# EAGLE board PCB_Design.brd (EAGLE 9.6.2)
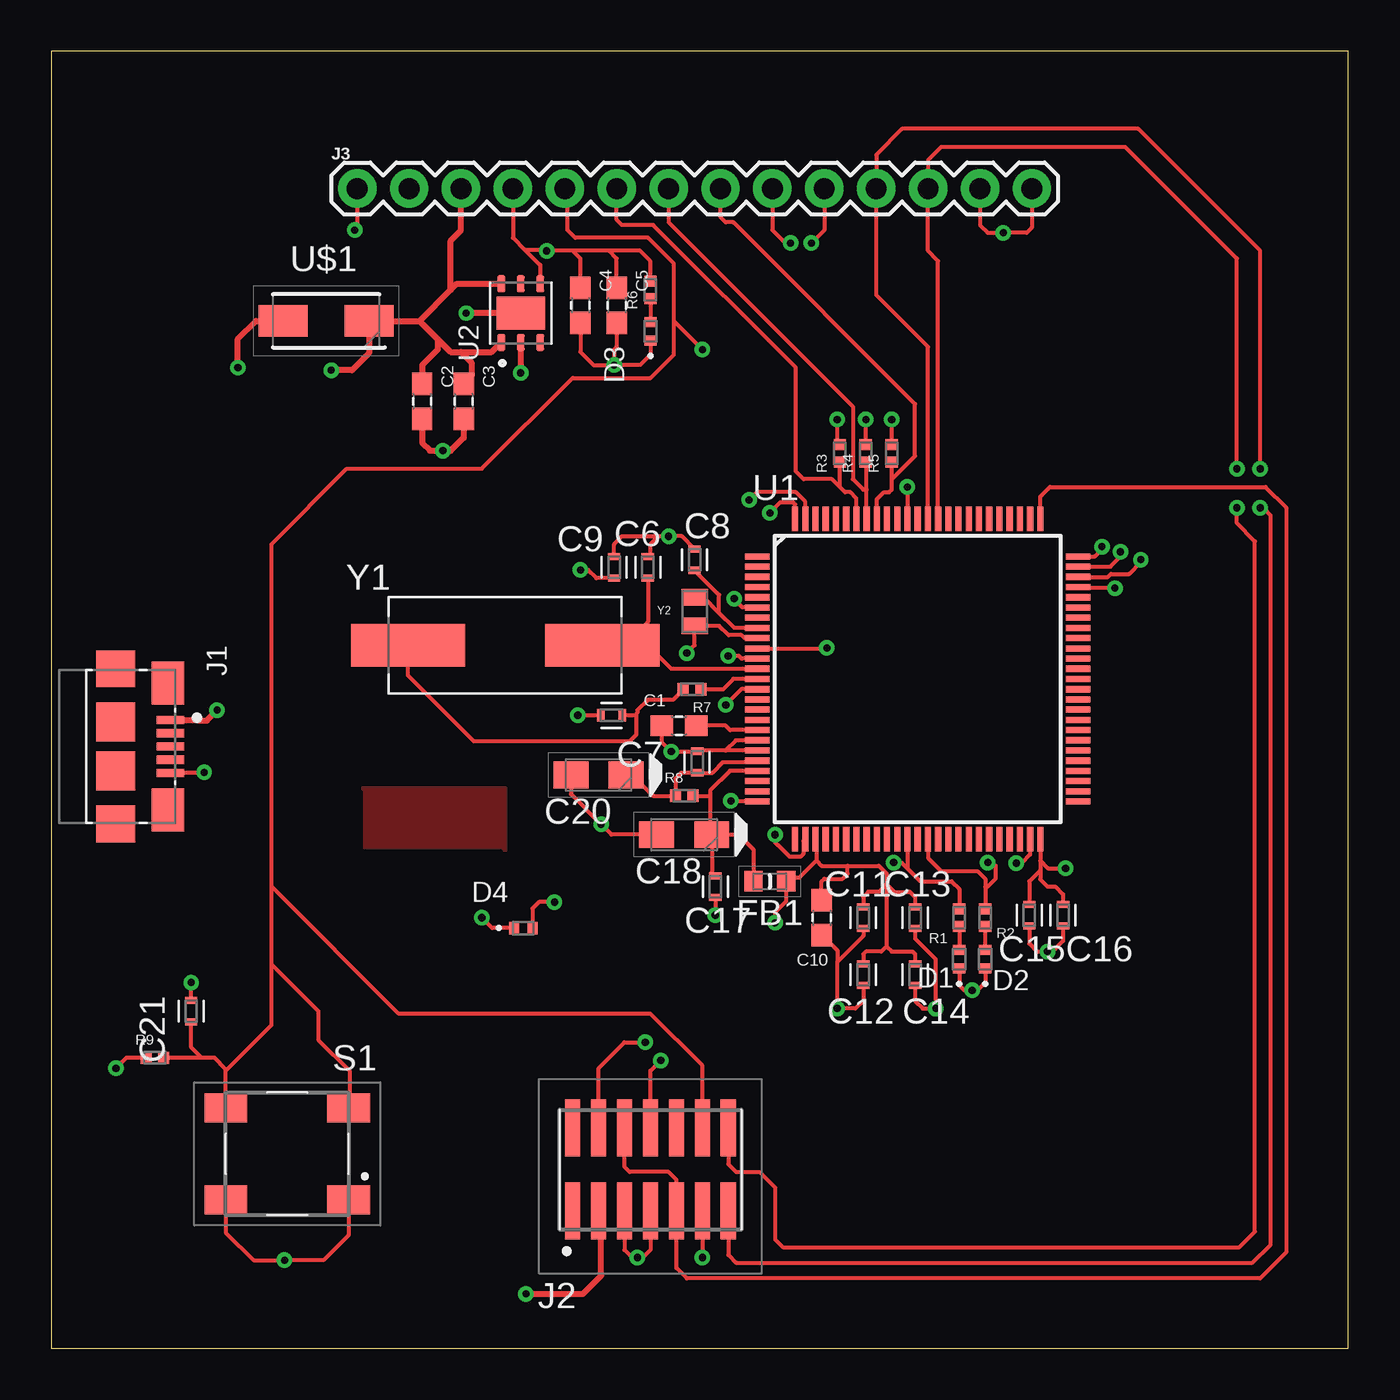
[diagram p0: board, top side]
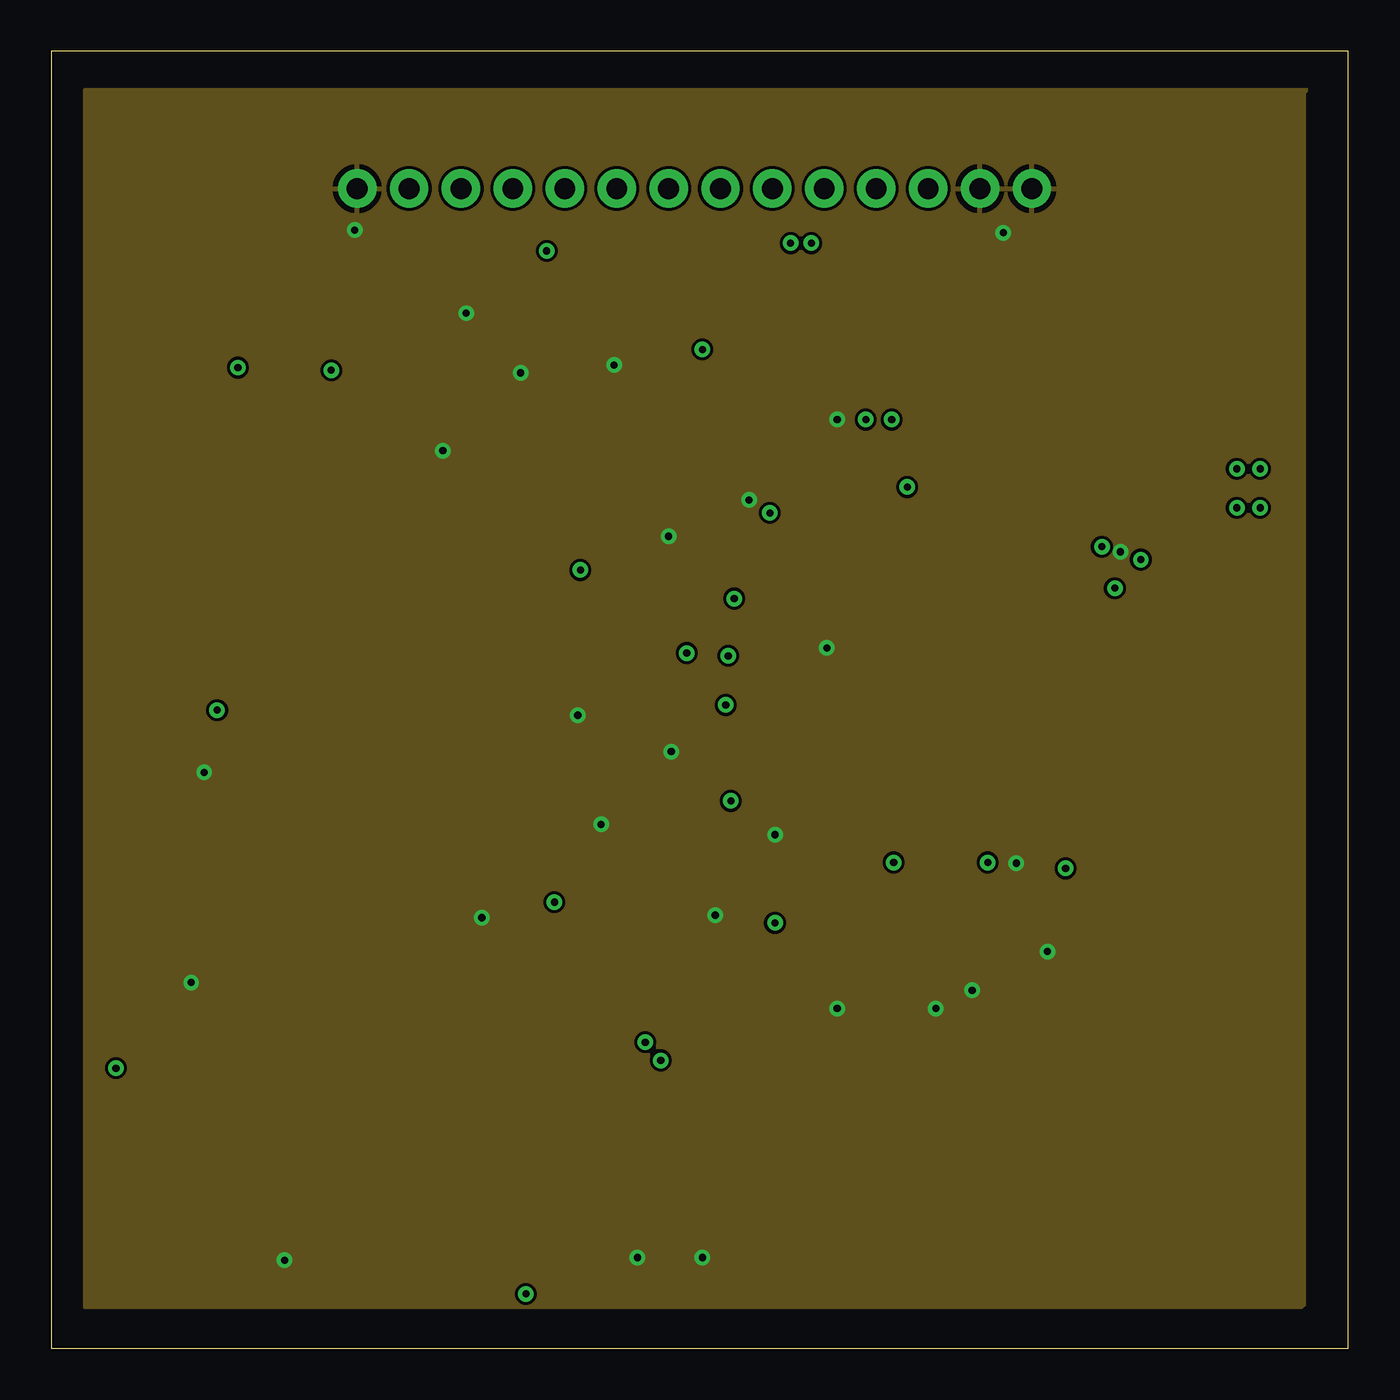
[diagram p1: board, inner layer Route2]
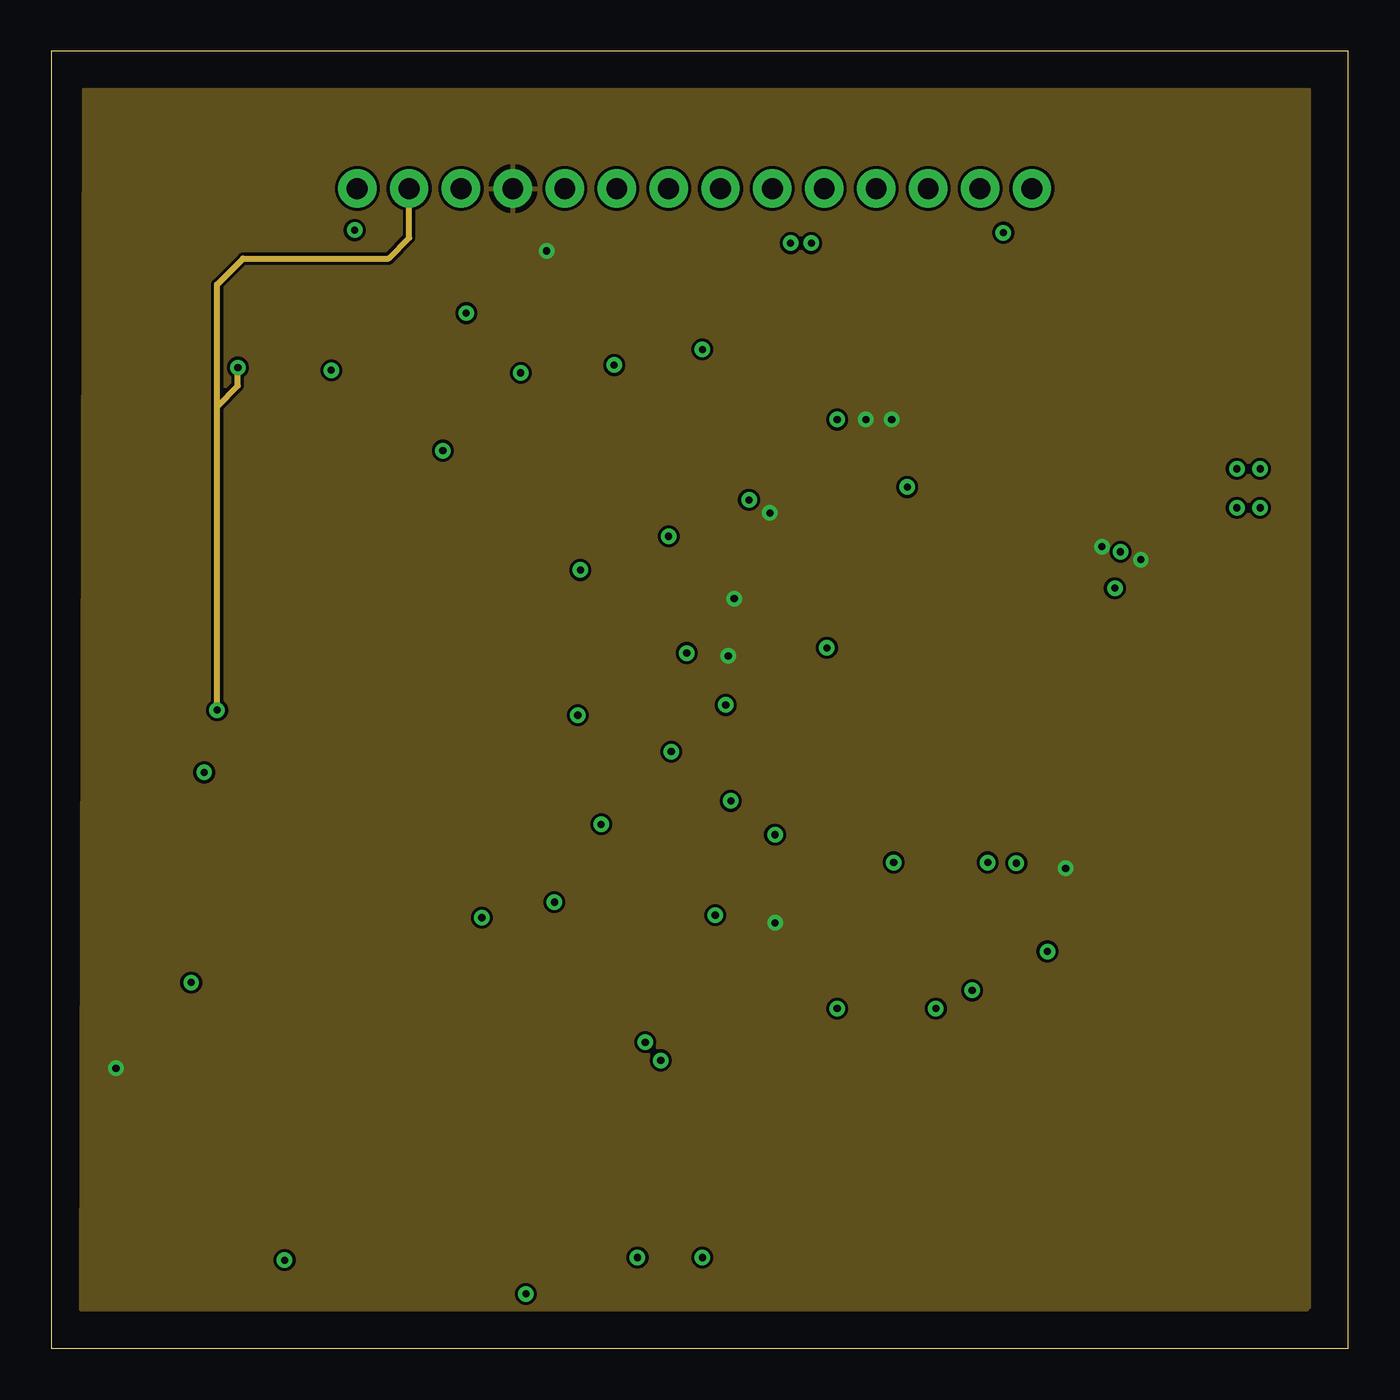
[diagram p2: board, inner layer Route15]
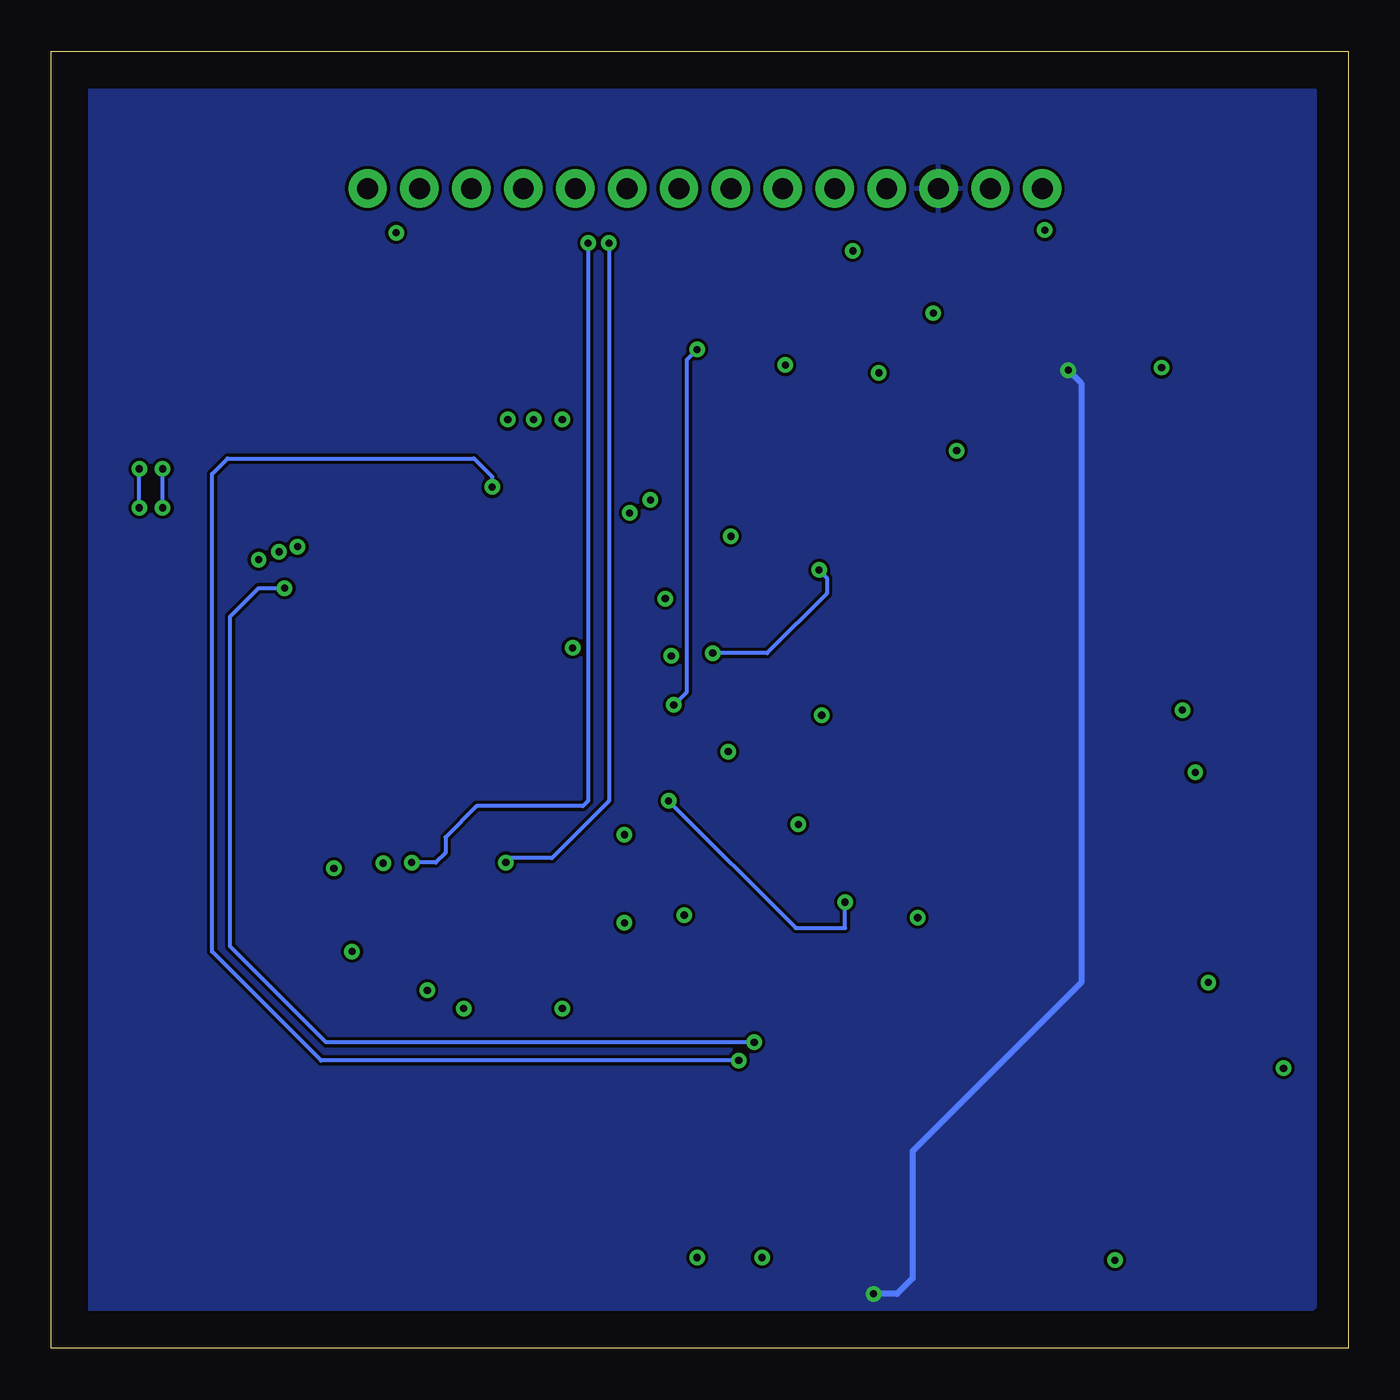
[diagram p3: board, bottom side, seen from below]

Size 63.5 x 63.5 mm. Coordinates in mm from the lower left corner, seen from the top.
Outline: 0,0 63.5,0 63.5,63.5 0,63.5 0,0
Copper layers (1+2*15+16): Top 0.035mm / dielectric 1.5mm / Route2 0.035mm / dielectric 0.15mm / Route15 0.035mm / dielectric 0.2mm / Bottom 0.035mm
Design rules "default *": minimum track width 8mil, minimum drill 0.35mm, track to track 6mil, track to pad 6mil, pad to pad 6mil, via to via 6mil, smd to smd 6mil, copper to edge 40mil, drill to drill 6mil, minimum pad ring 10mil, minimum via ring 8mil, stop-mask expansion 4mil, vias tented up to drill 0mil, thermal gap 10mil

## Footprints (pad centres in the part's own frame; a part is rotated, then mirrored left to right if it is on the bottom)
CAPC1608X90 = smd 1.1 x 1: 1 -0.85,0; 2 0.85,0
CAPC1005X55N = smd 0.35 x 0.6: 1 -0.525,0; 2 0.525,0
CAPPM3216X180N = smd 1.7 x 1.3: A -1.35,0; C 1.35,0
LED_SML-P11UTT86R = smd 0.5 x 0.6: A 0.45,0; C -0.45,0
BEADC1608X95N = smd 0.9 x 1: 1 -0.8,0; 2 0.8,0
AMPHENOL_10118192-0001LF = smd 0.4 x 1.35: 1 -1.3,0; 2 -0.65,0; 3 0,0; 4 0.65,0; 5 1.3,0 | smd 2.1 x 1.6: SH1 -3.1,-0.125; SH2 3.1,-0.125 | smd 1.8 x 1.9: SH3 -3.8,-2.675; SH6 3.8,-2.675 | smd 1.9 x 1.9: SH4 -1.2,-2.675; SH5 1.2,-2.675
FTSH10701LDVKA = smd 0.74 x 2.79: 1 -3.81,-2.035; 2 -3.81,2.035; 3 -2.54,-2.035; 4 -2.54,2.035; 5 -1.27,-2.035; 6 -1.27,2.035; 7 0,-2.035; 8 0,2.035; 9 1.27,-2.035; 10 1.27,2.035; 11 2.54,-2.035; 12 2.54,2.035; 13 3.81,-2.035; 14 3.81,2.035
1X14 = drill 1.016 pad 1.88: 1 0,0; 2 2.54,0; 3 5.08,0; 4 7.62,0; 5 10.16,0; 6 12.7,0; 7 15.24,0; 8 17.78,0; 9 20.32,0; 10 22.86,0; 11 25.4,0; 12 27.94,0; 13 30.48,0; 14 33.02,0
RESC1005X40N = smd 0.54 x 0.6: 1 -0.432,0; 2 0.432,0
LL3301FF065QJ = smd 2.1 x 1.4: 1 -3,2.25; 2 3,2.25; 3 -3,-2.25; 4 3,-2.25
LQFP100_14X14 = smd 1.2 x 0.3: 1 -7.85,6; 2 -7.85,5.5; 3 -7.85,5; 4 -7.85,4.5; 5 -7.85,4; 6 -7.85,3.5; 7 -7.85,3; 8 -7.85,2.5; 9 -7.85,2; 10 -7.85,1.5; 11 -7.85,1; 12 -7.85,0.5; 13 -7.85,0; 14 -7.85,-0.5; 15 -7.85,-1; 16 -7.85,-1.5; 17 -7.85,-2; 18 -7.85,-2.5; 19 -7.85,-3; 20 -7.85,-3.5; 21 -7.85,-4; 22 -7.85,-4.5; 23 -7.85,-5; 24 -7.85,-5.5; 25 -7.85,-6; 51 7.85,-6; 52 7.85,-5.5; 53 7.85,-5; 54 7.85,-4.5; 55 7.85,-4; 56 7.85,-3.5; 57 7.85,-3; 58 7.85,-2.5; 59 7.85,-2; 60 7.85,-1.5; 61 7.85,-1; 62 7.85,-0.5; 63 7.85,0; 64 7.85,0.5; 65 7.85,1; 66 7.85,1.5; 67 7.85,2; 68 7.85,2.5; 69 7.85,3; 70 7.85,3.5; 71 7.85,4; 72 7.85,4.5; 73 7.85,5; 74 7.85,5.5; 75 7.85,6 | smd 0.3 x 1.2: 26 -6,-7.85; 27 -5.5,-7.85; 28 -5,-7.85; 29 -4.5,-7.85; 30 -4,-7.85; 31 -3.5,-7.85; 32 -3,-7.85; 33 -2.5,-7.85; 34 -2,-7.85; 35 -1.5,-7.85; 36 -1,-7.85; 37 -0.5,-7.85; 38 0,-7.85; 39 0.5,-7.85; 40 1,-7.85; 41 1.5,-7.85; 42 2,-7.85; 43 2.5,-7.85; 44 3,-7.85; 45 3.5,-7.85; 46 4,-7.85; 47 4.5,-7.85; 48 5,-7.85; 49 5.5,-7.85; 50 6,-7.85; 76 6,7.85; 77 5.5,7.85; 78 5,7.85; 79 4.5,7.85; 80 4,7.85; 81 3.5,7.85; 82 3,7.85; 83 2.5,7.85; 84 2,7.85; 85 1.5,7.85; 86 1,7.85; 87 0.5,7.85; 88 0,7.85; 89 -0.5,7.85; 90 -1,7.85; 91 -1.5,7.85; 92 -2,7.85; 93 -2.5,7.85; 94 -3,7.85; 95 -3.5,7.85; 96 -4,7.85; 97 -4.5,7.85; 98 -5,7.85; 99 -5.5,7.85; 100 -6,7.85
SON95P300X300X100-7N = smd 0.84 x 0.4: 1 -1.435,0.95; 2 -1.435,0; 3 -1.435,-0.95; 4 1.435,-0.95; 5 1.435,0; 6 1.435,0.95 | smd 1.625 x 2.365: 7 0,0
DIOM5226X223N = smd 2.4 x 1.55: 1 -2.1,0; 2 2.1,0
XTAL_ABLS-8.000MHZ-B2-T = smd 5.6 x 2.1: 1 -4.75,0; 2 4.75,0
XTAL_ECS-.327-12.5-12QS-TR = smd 0.8 x 1.3: 1 -0.7,0; 2 0.7,0

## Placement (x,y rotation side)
C1  CC0603KRX5R7BB105  [CAPC1608X90]  30.73,30.48 0 top
C2  CC0603KRX5R7BB105  [CAPC1608X90]  18.16,46.35 270 top
C3  CC0603KRX5R7BB105  [CAPC1608X90]  20.19,46.35 270 top
C4  CC0603KRX5R7BB105  [CAPC1608X90]  25.91,51.05 270 top
C5  CC0603KRX5R7BB105  [CAPC1608X90]  27.69,51.05 270 top
C6  CC0402JRNPO9BN200  [CAPC1005X55N]  29.21,38.23 90 top
C7  CC0402JRNPO9BN200  [CAPC1005X55N]  27.43,30.99 180 top
C8  CC0402CRNPO9BN4R7  [CAPC1005X55N]  31.5,38.61 90 top
C9  CC0402CRNPO9BN4R7  [CAPC1005X55N]  27.56,38.23 90 top
C10  CC0603KRX5R7BB105  [CAPC1608X90]  37.72,21.08 270 top
C11  CC0402KRX7R7BB104  [CAPC1005X55N]  39.75,21.08 270 top
C12  CC0402KRX7R7BB104  [CAPC1005X55N]  39.75,18.29 270 top
C13  CC0402KRX7R7BB104  [CAPC1005X55N]  42.29,21.08 270 top
C14  CC0402KRX7R7BB104  [CAPC1005X55N]  42.29,18.29 270 top
C15  CC0402KRX7R7BB104  [CAPC1005X55N]  47.88,21.21 270 top
C16  CC0402KRX7R7BB104  [CAPC1005X55N]  49.53,21.21 270 top
C17  CC0402KRX7R7BB104  [CAPC1005X55N]  32.51,22.61 270 top
C18  TAJA105K016RNJ  [CAPPM3216X180N]  30.99,25.15 180 top
C19  CC0402KRX7R7BB104  [CAPC1005X55N]  31.62,28.7 90 top
C20  TAJA105K016RNJ  [CAPPM3216X180N]  26.8,28.07 180 top
C21  CC0402KRX7R7BB104  [CAPC1005X55N]  6.86,16.51 90 top
D1  SML-P12MTT86  [LED_SML-P11UTT86R]  44.45,19.05 90 top
D2  SML-P12MTT86  [LED_SML-P11UTT86R]  45.72,19.05 90 top
D3  SML-P12VTT86  [LED_SML-P11UTT86R]  29.34,49.78 90 top
D4  SML-P12MTT86  [LED_SML-P11UTT86R]  23.11,20.57 0 top
FB1  BK1608HS601-T  [BEADC1608X95N]  35.18,22.86 0 top
J1  10118192-0001LF  [AMPHENOL_10118192-0001LF]  5.84,29.46 270 top
J2  FTSH-107-01-L-DV-K-A  [FTSH10701LDVKA]  29.34,8.76 0 top
J3  [1X14]  14.99,56.77 0 top
R1  RC0402FR-071KL  [RESC1005X40N]  44.45,21.08 90 top
R2  RC0402FR-071KL  [RESC1005X40N]  45.72,21.08 90 top
R3  RC0402FR-071KL  [RESC1005X40N]  38.61,43.81 90 top
R4  RC0402FR-071KL  [RESC1005X40N]  39.88,43.81 90 top
R5  RC0402FR-071KL  [RESC1005X40N]  41.15,43.81 90 top
R6  RC0402FR-071KL  [RESC1005X40N]  29.34,51.82 90 top
R7  RC0402FR-071KL  [RESC1005X40N]  31.37,32.26 180 top
R8  RC0402FR-071KL  [RESC1005X40N]  30.99,27.05 0 top
R9  RC0402FR-071KL  [RESC1005X40N]  5.08,14.22 0 top
S1  LL3301FF065QJ  [LL3301FF065QJ]  11.56,9.53 180 top
U1  STM32L476VCT6  [LQFP100_14X14]  42.42,32.77 0 top
U2  LD39050PU33R  [SON95P300X300X100-7N]  22.99,50.67 90 top
U$1  STPS1L30A  [DIOM5226X223N]  13.46,50.29 180 top
Y1  ABLS-8.000MHZ-B2-T  [XTAL_ABLS-8.000MHZ-B2-T]  22.23,34.42 0 top
Y2  ECS-.327-12.5-12QS-TR  [XTAL_ECS-.327-12.5-12QS-TR]  31.5,36.07 90 top

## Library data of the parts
C1-C5 C10 = ce-capstone; DESCRIPTION: 1µF ±10% 16V Ceramic Capacitor X5R 0603 _1608 Metric_; DIGI-KEY_PART_NUMBER: 311-1444-1-ND; DIGI-KEY_PURCHASE_URL: https://www.digikey.com/product-detail/en/yageo/CC0603KRX5R7BB105/311-1444-1-ND/2833750?utm_source=snapeda&utm_medium=aggregator&utm_campaign=symbol; MF: Yageo; MP: CC0603KRX5R7BB105; PACKAGE: 0603 Yageo
C6 C7 = ce-capstone; DESCRIPTION: 20pF ±5% 50V Ceramic Capacitor C0G, NP0 0402 _1005 Metric_; DIGI-KEY_PART_NUMBER: 311-1417-1-ND; DIGI-KEY_PURCHASE_URL: https://www.digikey.com/product-detail/en/yageo/CC0402JRNPO9BN200/311-1417-1-ND/2833723?utm_source=snapeda&utm_medium=aggregator&utm_campaign=symbol; MF: Yageo; MP: CC0402JRNPO9BN200; PACKAGE: 0402 Yageo
C8 C9 = ce-capstone; DESCRIPTION: 4.7pF ±0.25pF 50V Ceramic Capacitor C0G, NP0 0402 _1005 Metric_; DIGI-KEY_PART_NUMBER: 311-1367-1-ND; DIGI-KEY_PURCHASE_URL: https://www.digikey.com/product-detail/en/yageo/CC0402CRNPO9BN4R7/311-1367-1-ND/2103151?utm_source=snapeda&utm_medium=aggregator&utm_campaign=symbol; MF: Yageo; MP: CC0402CRNPO9BN4R7; PACKAGE: 0402 Yageo
C11-C17 C19 C21 = ce-capstone; DESCRIPTION: 0.1µF ±10% 16V Ceramic Capacitor X7R 0402 _1005 Metric_; DIGI-KEY_PART_NUMBER: 311-1338-1-ND; DIGI-KEY_PURCHASE_URL: https://www.digikey.com/product-detail/en/yageo/CC0402KRX7R7BB104/311-1338-1-ND/2103122?utm_source=snapeda&utm_medium=aggregator&utm_campaign=symbol; MF: Yageo; MP: CC0402KRX7R7BB104; PACKAGE: 0402 Yageo
C18 C20 = ce-capstone; ALLIED_NUMBER: 70474975; ALLIED_PRICE-STOCK: https://www.alliedelec.com/avx-taja105k016r/70474975/; DESCRIPTION: Capacitor tantalum TAJ 1206 1uF 16V AVX 1uF SMD Solid MnO2 Tantalum Electrolytic Capacitor, 16 V dc +/-10%, TAJ Series; HEIGHT: 1.8mm; MANUFACTURER_NAME: AVX; MANUFACTURER_PART_NUMBER: TAJA105K016RNJ; MOUSER_PART_NUMBER: 581-TAJA105K016RNJ; MOUSER_PRICE-STOCK: https://www.mouser.com/Search/Refine.aspx?Keyword=581-TAJA105K016R; RS_PART_NUMBER: 6992804P; RS_PRICE-STOCK: http://uk.rs-online.com/web/p/products/6992804P
D1 D2 D4 = ce-capstone; AVAILABILITY: Unavailable; DESCRIPTION: Green 572nm LED Indication - Discrete 2V 0402 _1006 Metric_; MF: Rohm; MP: SML-P12MTT86; PACKAGE: 0402 Rohm; PRICE: None
D3 = ce-capstone; AVAILABILITY: Unavailable; DESCRIPTION: Red 630nm LED Indication - Discrete 2V 0402 _1006 Metric_; MF: Rohm; MP: SML-P12VTT86; PACKAGE: 0402 Rohm; PRICE: None
FB1 = ce-capstone; DESCRIPTION: Ferrite Chip Bead(Lead Free); HEIGHT: 0.95mm; MANUFACTURER_NAME: Taiyo Yuden; MANUFACTURER_PART_NUMBER: BK1608HS601-T
J1 = ce-capstone; AVAILABILITY: Unavailable; DESCRIPTION: USB - micro B USB 2.0 Receptacle Connector 5 Position Surface Mount, Right Angle; MF: Amphenol ICC; MP: 10118192-0001LF; PACKAGE: None; PRICE: None
J2 = ce-capstone; DESCRIPTION: Headers & Wire Housings .050" Micro Terminal Strip; HEIGHT: 5.97mm; MANUFACTURER_NAME: SAMTEC; MANUFACTURER_PART_NUMBER: FTSH-107-01-L-DV-K-A; MOUSER_PART_NUMBER: 200-FTSH10701LDVKA; MOUSER_PRICE-STOCK: https://www.mouser.com/Search/Refine.aspx?Keyword=200-FTSH10701LDVKA
J3 = SparkFun-Connectors
R1-R9 = ce-capstone; DESCRIPTION: 510 Ohms ±1% 0.063W, 1/16W Chip Resistor 0402 _1005 Metric_ Moisture Resistant Thick Film; DIGI-KEY_PART_NUMBER: 311-510LRCT-ND; DIGI-KEY_PURCHASE_URL: https://www.digikey.com/product-detail/en/yageo/RC0402FR-07510RL/311-510LRCT-ND/729579?utm_source=snapeda&utm_medium=aggregator&utm_campaign=symbol; MF: Yageo; MP: RC0402FR-07510RL; PACKAGE: 1005 Panasonic Electronic Components
S1 = ce-capstone; DESCRIPTION: Pushbutton Switches 50mA 12VDC F065 7.0mm J-Lead; HEIGHT: 7.3mm; MANUFACTURER_NAME: E-Switch; MANUFACTURER_PART_NUMBER: LL3301FF065QJ; MOUSER_PART_NUMBER: 612-LL3301FF065QJ; MOUSER_PRICE-STOCK: https://www.mouser.com/Search/Refine.aspx?Keyword=612-LL3301FF065QJ
U1 = ce-capstone; FARNELL: 2518171; FLASH: 256kB; SRAM: 128kB
U2 = ce-capstone; AVAILABILITY: Unavailable; DESCRIPTION: Linear Voltage Regulator IC 1 Output 500mA 6-DFN _3x3_; MF: STMicroelectronics; MP: LD39050PU33R; PACKAGE: DFN-6 STMicroelectronics; PRICE: None
U$1 = ce-capstone
Y1 = ce-capstone; AVAILABILITY: Unavailable; DESCRIPTION: 8MHz ±20ppm Crystal 18pF 80 Ohms HC-49/US; MF: Abracon LLC; MP: ABLS-8.000MHZ-B2; PACKAGE: HC-49/US Abracon LLC; PRICE: None
Y2 = ce-capstone; AVAILABILITY: Unavailable; DESCRIPTION: 32.768kHz ±20ppm Crystal 12.5pF 90 kOhms 2-SMD, No Lead; MF: ECS Inc.; MP: ECS-.327-12.5-12QS-TR; PACKAGE: SMD-2 ECS International; PRICE: None

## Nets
3V3: C4.1 C5.1 C10.1 C11.1 C12.1 C13.1 C14.1 C15.1 C16.1 FB1.2 J3.4 R4.2 R5.2 R6.2 R9.1 U1.6 U1.11 U1.28 U1.50 U1.73 U1.75 U1.100 U2.4
5V: C2.1 C3.1 J2.3 J3.3 U2.1 U2.6 U$1.1
5V_IN: J1.1 J3.2 U$1.2
BOOT0: J3.6 R3.1 U1.94
GND: C1.1 C2.2 C3.2 C4.2 C5.2 C6.2 C7.2 C8.2 C9.2 C10.2 C11.2 C12.2 C13.2 C14.2 C15.2 C16.2 C17.2 C18.C C19.2 C20.C C21.2 D1.C D2.C D3.C D4.C J1.5 J2.5 J2.7 J2.11 J3.1 J3.13 J3.14 R3.2 S1.1 S1.2 U1.10 U1.19 U1.20 U1.27 U1.49 U1.74 U1.99 U2.2 U2.7
I2C1_SCL: J3.8 R5.1 U1.92
I2C1_SDA: J3.7 R4.1 U1.93
LED-G: D2.A R2.1
LED-R: D1.A R1.1
LED_G: J3.10 R2.2 U1.39
LED_R: J3.9 R1.2 U1.37
N$1: D4.A U1.25
N$9: C7.1 R7.2 Y1.1
N$11: C1.2 U1.18
N$14: D3.A R6.1
NRST: C21.1 J2.12 J3.5 R9.2 S1.3 S1.4 U1.14
PC14-OSC32-IN: C8.1 U1.8 Y2.2
PC15-OSC32-OUT: C9.1 U1.9 Y2.1
PH0-OSC-IN: C6.1 U1.12 Y1.2
PH1-OSC-OUT: R7.1 U1.13
SWCLK: J2.6 J2.9 U1.76
SWDIO: J2.4 U1.72
SWO: J2.8 U1.89
USART_RX: J2.13 J3.11 U1.87
USART_TX: J2.14 J3.12 U1.86
VDDA: C17.1 C18.A FB1.1 R8.2 U1.22
VREF_PLUS: C19.1 C20.A R8.1 U1.21

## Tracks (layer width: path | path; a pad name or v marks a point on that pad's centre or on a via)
3V3  (via drill 0.35)
  Top 0.203: 37.47,23.88 36.64,23.05 36.17,23.05 FB1.2 35.98,21.88 35.43,21.34 v35.43,20.83 | 37.47,23.88 37.47,24.64 37.42,24.68 U1.28 | U1.50 48.42,23.88 | 48.42,23.88 48.42,23.4 | 48.42,23.4 47.88,22.86 C15.1 | 48.42,23.4 48.42,22.96 48.77,22.61 49.15,22.61 49.53,22.23 C16.1 | 37.47,23.88 37.72,23.62 38.99,23.62 | 40.89,22.73 40.89,23.24 40.51,23.62 38.99,23.62 | 40.89,22.73 40.51,22.35 40.01,22.35 39.75,22.1 C11.1 | 40.89,22.73 41.27,22.35 42.04,22.35 42.29,22.1 C13.1 | 40.89,22.73 40.89,19.68 | 40.89,19.68 40.64,19.43 39.88,19.43 39.75,19.3 C12.1 | 40.89,19.68 41.15,19.43 42.16,19.43 42.29,19.3 C14.1 | C10.1 37.72,22.86 37.85,22.99 38.73,22.99 38.99,23.24 38.99,23.62 | R4.2 v39.88,45.47 | R5.2 v41.15,45.47 | 48.42,23.88 48.8,23.5 v49.66,23.5 | J3.4 22.61,54.36 23.18,53.78 | U2.4 23.94,53.02 23.18,53.78 | 23.18,53.78 24.19,53.78 v24.26,53.72 25.53,53.72 | C4.1 25.91,53.34 25.53,53.72 | C5.1 27.69,53.34 27.3,53.72 | 27.3,53.72 25.53,53.72 | R6.2 29.34,53.21 28.83,53.72 27.3,53.72 | R9.1 3.68,14.22 v3.17,13.72 | U1.75 51.09,38.77 51.44,39.12 v51.44,39.24 | U1.73 51.73,37.77 51.88,37.91 52.77,37.91 53.34,38.48 v53.34,38.61 | U1.6 33.84,36.27 33.44,36.67 v33.44,36.7 | U1.11 33.8,33.77 33.67,33.9 v33.15,33.9 | U1.100 36.42,41.31 36.32,41.4 35.69,41.4 v35.18,40.89
  pour Route15: 1.46,1.91 61.47,1.91 61.59,2.03 61.59,61.59 1.59,61.59
5V  (via drill 0.35)
  Top 0.305: 18.03,50.29 U$1.1 15.56,48.71 14.73,47.88 v13.72,47.88 | J3.3 20.07,54.74 19.56,54.23 19.56,51.82 | 18.03,50.29 19.56,51.82 | 19.56,51.82 19.85,52.11 U2.6 | 18.03,50.29 18.92,49.4 | 18.92,49.4 18.92,48.9 18.16,48.13 C2.1 | 18.92,49.4 19.56,48.77 20.07,48.77 | U2.1 21.57,48.77 20.07,48.77 | 20.07,48.77 20.57,48.26 20.57,47.59 C3.1 | v23.24,2.67 26.04,2.67 26.92,3.56 26.92,6.6 J2.3
  Bottom 0.305: v13.72,47.88 13.08,47.24 13.08,17.91 21.34,9.65 21.34,3.43 22.1,2.67 v23.24,2.67
  pour Bottom: 1.65,61.59 1.65,2.03 1.78,1.91 61.59,1.91 61.59,61.59
5V_IN  (via drill 0.35)
  Top 0.305: J1.1 7.21,30.76 7.24,30.73 7.62,30.73 v8.13,31.24 | v9.14,48.01 9.14,49.4 10.03,50.29 U$1.2
  Route15 0.305: v8.13,31.24 8.13,46.1 | 8.13,46.1 8.13,49.15 8.13,52.07 9.4,53.34 16.51,53.34 17.53,54.36 J3.2 | 8.13,46.1 9.14,47.12 v9.14,48.01
BOOT0
  Top 0.203: U1.94 39.42,41.61 39.12,41.91 38.86,41.91 38.61,42.16 | 38.61,42.16 R3.1 | 38.61,42.16 38.23,42.55 36.83,42.55 36.45,42.93 36.45,48.01 29.46,54.99 27.94,54.99 27.69,55.24 J3.6
GND  (via drill 0.35)
  Top 0.203: J1.5 5.87,28.19 v7.49,28.19 | U1.20 33.02,29.27 | 33.02,29.27 31.66,29.27 C19.2 31.62,29.21 v30.35,29.21 29.88,29.68 C1.1 | U1.19 33.52,29.77 33.02,29.27 | C20.C 25.45,27.13 v26.92,25.65 27.43,25.15 C18.C | C17.2 v32.51,21.21 | C13.2 42.29,20.07 43.31,19.05 v43.31,16.64 42.67,16.64 42.29,17.02 C14.2 | C11.2 39.75,20.19 38.48,18.92 | 38.48,18.92 v38.48,16.64 39.37,16.64 39.75,17.02 C12.2 | C15.2 47.88,19.81 48.26,19.43 v48.77,19.43 49.02,19.43 49.53,19.94 C16.2 | U1.49 47.92,24.17 47.5,23.75 v47.24,23.75 | C10.2 38.48,19.47 38.48,18.92 | D1.C 44.45,17.78 44.7,17.53 v45.09,17.53 45.34,17.53 45.72,17.91 D2.C | C7.2 v25.78,30.99 | C8.2 30.88,39.75 v30.23,39.75 29.72,39.75 | C6.2 29.34,38.88 29.34,39.37 29.72,39.75 | C9.2 27.56,39.37 27.94,39.75 29.72,39.75 | D3.C 29.34,48.64 28.83,48.13 v27.56,48.13 | C5.2 27.69,49.02 27.56,48.9 v27.56,48.13 | C4.2 25.91,48.77 26.54,48.13 v27.56,48.13 | S1.2 8.56,5.67 9.91,4.32 v11.43,4.32 13.34,4.32 14.56,5.54 S1.1 | C21.2 v6.86,17.91 | J2.5 28.07,4.83 28.45,4.45 v28.7,4.45 28.96,4.45 29.34,4.83 J2.7 | J2.11 v31.88,4.45 | J3.13 45.47,54.99 45.85,54.61 v46.61,54.61 47.75,54.61 48.01,54.86 J3.14 | U1.74 51.85,38.27 52.34,38.76 v52.34,38.99 | v14.86,54.74 14.99,54.86 J3.1 | U1.10 37.7,34.27 37.72,34.29 v37.97,34.29 | U1.99 36.92,41.44 36.45,41.91 34.54,41.91 v34.16,41.53 | U1.27 36.82,24.82 36.82,24.21 36.67,24.06 36.16,24.06 35.59,24.64 35.56,24.64 35.43,24.77 v35.43,25.15 | R3.2 38.48,44.37 v38.48,45.47 | D4.C 21.59,20.57 v21.08,21.08
  Top 0.305: C2.2 18.16,44.32 18.54,43.94 v19.18,43.94 19.56,43.94 20.19,44.58 C3.2 | U2.2 v22.99,47.75 | U2.7 v20.32,50.67
  pour Route2: 1.65,61.59 1.65,2.03 61.21,2.03 61.34,2.16 61.34,61.47 61.47,61.59
  pour Top: 15.24,27.43 22.23,27.43 22.23,24.38 22.1,24.51 15.37,24.51 15.37,27.3
I2C1_SCL
  Top 0.203: U1.92 40.42,41.56 40.77,41.91 41.02,41.91 41.15,42.04 41.15,42.42 41.15,42.55 | 41.15,42.55 R5.1 | 41.15,42.55 42.29,43.69 42.29,46.23 33.4,55.12 33.02,55.12 32.77,55.37 J3.8
I2C1_SDA
  Top 0.203: U1.93 39.92,42.04 | 39.92,42.04 39.92,43.34 R4.1 | J3.7 30.23,55.12 39.24,46.1 39.24,42.55 39.75,42.04 39.92,42.04
LED-G
  Top 0.203: D2.A R2.1
LED-R
  Top 0.203: R1.1 D1.A
LED_G  (via drill 0.35)
  Top 0.203: U1.39 42.92,24.01 43.56,23.37 45.34,23.37 45.72,22.99 45.72,22.61 | 45.72,22.61 R2.2 | J3.10 37.85,54.74 v37.21,54.1 | v45.85,23.79 46.06,23.79 46.23,23.62 46.23,22.99 45.85,22.61 45.72,22.61
  Bottom 0.203: v37.21,54.1 37.21,26.8 37.47,26.54 42.67,26.54 44.2,25.02 44.2,24.26 44.67,23.79 v45.85,23.79
LED_R  (via drill 0.35)
  Top 0.203: U1.37 41.92,23.49 | R1.2 44.45,22.48 44.07,22.86 42.55,22.86 41.92,23.49 | J3.9 35.31,54.74 35.94,54.1 v36.2,54.1 | v41.24,23.79 41.62,23.79 41.92,23.49
  Bottom 0.203: v36.2,54.1 36.2,26.8 38.99,24 41.03,24 v41.24,23.79
N$1  (via drill 0.35)
  Top 0.203: U1.25 33.3,26.77 v33.27,26.8 | v24.64,21.84 23.88,21.84 23.56,21.53 D4.A
  Bottom 0.203: v33.27,26.8 27.05,20.57 24.64,20.57 v24.64,21.84
N$9
  Top 0.203: R7.2 30.43,31.75 29.21,31.75 28.7,31.24 28.7,31.11 28.64,31.05 | 28.64,31.05 28.57,30.99 C7.1 | 28.64,31.05 28.64,30.04 28.32,29.72 20.7,29.72 17.48,32.94 Y1.1
N$11
  Top 0.203: U1.18 33.23,30.27 33.02,30.48 C1.2
N$14
  Top 0.203: R6.1 D3.A
NRST  (via drill 0.35)
  Top 0.203: S1.4 8.56,13.59 | 8.56,13.59 8.56,13.67 8,14.22 7.37,14.22 | 7.37,14.22 R9.2 | 7.37,14.22 6.86,14.73 C21.1 | S1.3 14.61,11.82 14.61,13.59 13.08,15.11 13.08,16.51 10.79,18.8 | 8.56,13.59 10.79,15.83 10.79,18.8 | 10.79,18.8 10.79,22.61 | 10.79,22.61 10.79,39.37 14.48,43.05 21.08,43.05 25.53,47.5 29.34,47.5 30.48,48.64 30.48,50.29 | 30.48,50.29 30.48,53.09 29.21,54.36 25.65,54.36 25.27,54.74 25.27,56.64 J3.5 | J2.12 31.88,13.84 29.34,16.38 17.02,16.38 10.79,22.61 | U1.14 33.79,32.27 v33.02,31.5 | v31.88,48.9 30.48,50.29
  Bottom 0.203: v33.02,31.5 32.38,32.13 32.38,48.39 v31.88,48.9
PC14-OSC32-IN
  Top 0.203: U1.8 33.44,35.27 32.7,36.01 | Y2.2 31.94,36.77 32.7,36.01 | 32.7,36.01 32.7,36.88 C8.1
PC15-OSC32-OUT  (via drill 0.35)
  Top 0.203: C9.1 26.69,37.7 26.29,38.1 v25.91,38.1 | v31.11,34.04 31.5,34.42 Y2.1 32.7,35.37 33.16,34.91 33.8,34.91 33.94,34.77 U1.9
  Bottom 0.203: v25.91,38.1 25.53,37.72 25.53,36.96 28.45,34.04 v31.11,34.04
PH0-OSC-IN
  Top 0.203: U1.12 30.36,33.27 29.08,34.54 28.19,34.54 | Y1.2 27.1,34.54 28.19,34.54 | C6.1 29.21,35.56 28.19,34.54
PH1-OSC-OUT
  Top 0.203: R7.1 32.89,32.26 33.4,32.77 U1.13
SWCLK
  Top 0.203: U1.76 48.42,41.69 48.9,42.16 59.44,42.16 60.45,41.15 60.45,4.7 59.18,3.43 31.11,3.43 30.61,3.94 J2.9 30.61,8.26 30.23,8.64 28.32,8.64 28.07,8.89 J2.6
SWDIO  (via drill 0.35)
  Top 0.203: J2.4 26.8,13.72 28.07,14.99 v29.08,14.99 | v52.07,37.21 50.32,37.21 U1.72
  Bottom 0.203: v29.08,14.99 50.04,14.99 54.74,19.68 54.74,35.81 53.34,37.21 v52.07,37.21
SWO  (via drill 0.35)
  Top 0.203: v41.91,42.16 v41.92,42.16 U1.89 | J2.8 29.34,13.59 v29.84,14.1
  Bottom 0.203: v29.84,14.1 50.29,14.1 55.63,19.43 55.63,42.8 54.86,43.56 42.8,43.56 41.91,42.67 v41.91,42.16
USART_RX  (via drill 0.35)
  Top 0.203: U1.87 42.92,49.03 40.39,51.56 J3.11 40.39,58.42 41.66,59.69 53.21,59.69 59.18,53.72 v59.18,43.05 | J2.13 33.15,4.57 33.53,4.19 58.8,4.19 59.69,5.08 59.69,40.77 59.31,41.15 v59.18,41.15
  Bottom 0.203: v59.18,41.15 v59.18,43.05
USART_TX  (via drill 0.35)
  Top 0.203: U1.86 43.42,53.23 42.93,53.72 J3.12 42.93,58.17 43.56,58.8 52.58,58.8 58.04,53.34 v58.04,43.05 | J2.14 33.15,9.02 33.53,8.64 34.67,8.64 35.43,7.87 35.43,5.33 35.81,4.95 58.17,4.95 58.93,5.71 58.93,39.5 58.04,40.39 v58.04,41.15
  Bottom 0.203: v58.04,41.15 v58.04,43.05
VDDA
  Top 0.203: U1.22 33.22,28.27 32.26,27.3 32.26,27.05 | 32.26,27.05 32.26,25.23 C18.A | R8.2 32.26,27.05 | C18.A 32.34,23.3 C17.1 | C18.A 33.66,25.15 34.38,24.42 FB1.1
VREF_PLUS
  Top 0.203: U1.21 34.5,28.7 32.89,28.7 32.37,28.18 C19.1 30.84,28.18 30.56,27.89 R8.1 29.46,27.05 28.45,28.07 C20.A

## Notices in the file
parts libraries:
SparkFun-Connectors: Licensing: Creative Commons ShareAlike 4.0 International - https://creativecommons.org/licenses/by-sa/4.0
